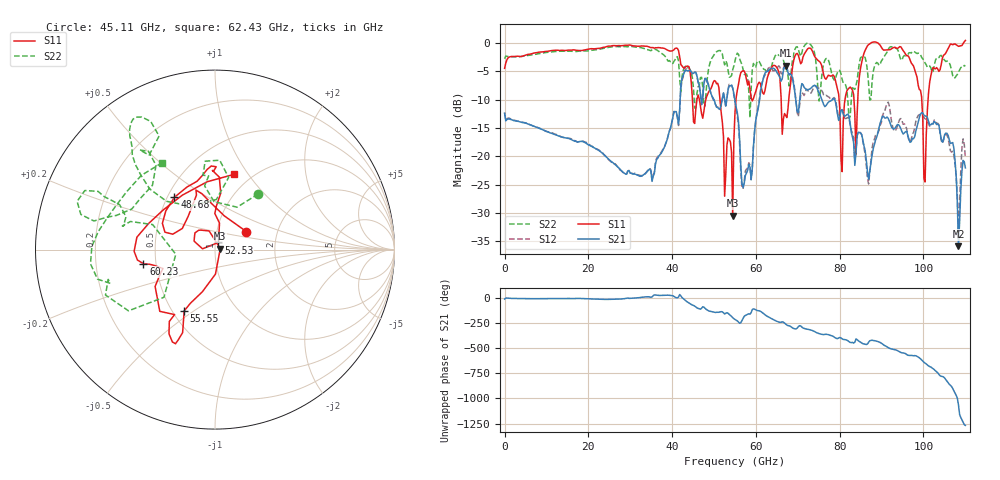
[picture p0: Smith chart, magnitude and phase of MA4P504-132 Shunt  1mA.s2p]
!Keysight Technologies,N5247B,US61255204,A.15.70.20
!Date: Friday, October 21, 2022 14:55:33
!Correction: S11(C  4-Port  )
!S31(C  4-Port  )
!S13(C  4-Port  )
!S33(C  4-Port  )
!S2P File: Measurements: S11, S31, S13, S33:
# Hz S  dB  R 50
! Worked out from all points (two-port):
!   401 points, 10 MHz to 110 GHz, reference 50 ohm
!   highest |S21| = -4.01 dB at 67.1 GHz (marker M1); lowest = -35.9 dB at 108.4 GHz (marker M2)
!   |S21| within 3 dB of the highest: 42.16 GHz to 46.25 GHz (4.099 GHz wide, 9.27 % of centre); 61.52 GHz to 68.91 GHz (7.396 GHz wide, 11.3 % of centre)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
!   lowest |S11| = -30.5 dB at 54.46 GHz (marker M3), VSWR 1.06, Z = 53 + j0.577 ohm
!   |S11| at or under -10 dB: 46.51 GHz to 48.04 GHz (1.53 GHz wide, 3.24 % of centre); 51.43 GHz to 55.24 GHz (3.815 GHz wide, 7.15 % of centre); 66.02 GHz to 67.84 GHz (1.818 GHz wide, 2.72 % of centre)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
!   |S22| runs from -13.3 to 0.0 dB; largest |S21 - S12| = 0.24
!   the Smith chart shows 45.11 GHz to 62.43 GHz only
!   S11 on the Smith chart (normalised r, x): 45.11 GHz: 1.39, +0.29; 48.68 GHz: 0.54, +0.37; 52.53 GHz: 1.04, +0.08; 55.55 GHz: 0.57, -0.46; 60.23 GHz: 0.43, -0.08; 62.43 GHz: 0.84, +0.86
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1e7  -4.46 -176.7  -12.37 -9.5  -12.35 -9.4  -2.78 -176.8
1.843332e10  -1.32 118.1  -17.37 -4.3  -17.39 -4.2  -1.41 124.6
3.685665e10  -0.80 115.3  -19.92 26.5  -19.76 26.5  -1.47 122.2
4.51059e10  -13.92 29.9  -5.36 -73.2  -5.44 -72.3  -8.12 52.2
4.868058e10  -8.66 127.8  -7.49 -126.1  -7.33 -124.8  -4.64 134.9
5.253022e10  -27.05 64.0  -9.85 -158.4  -9.96 -158.7  -3.85 124.8
5.445505e10  -30.47 10.5  -7.92 165.1  -8.01 164.2  -4.71 160.9
5.5005e10  -12.19 -106.7  -10.21 146.9  -10.45 145.0  -3.19 166.7
5.555495e10  -8.34 -116.7  -12.29 133.1  -12.88 132.3  -1.79 160.7
5.72048e10  -4.93 -114.8  -24.77 178.9  -24.40 -170.9  -5.54 159.8
6.022952e10  -7.83 -168.8  -12.56 -122.3  -12.35 -117.7  -3.42 -165.8
6.242932e10  -7.27 75.6  -5.05 -174.0  -5.25 -167.8  -4.94 121.2
6.71039e10  -12.78 -42.0  -4.01 101.5  -3.69 101.8  -4.38 45.6
7.342832e10  -1.33 138.5  -7.74 37.7  -8.45 35.9  -0.67 108.4
8.112762e10  -10.66 -29.9  -12.95 -53.1  -13.26 -54.0  -7.15 -124.7
8.525225e10  -3.37 38.3  -16.14 -87.7  -16.25 -86.5  -2.45 -23.7
9.185165e10  -1.17 90.5  -13.78 -139.2  -11.12 -133.5  -0.79 83.8
9.872602e10  -7.41 152.7  -13.97 132.9  -12.79 132.5  -1.78 177.4
1.003759e11  -24.53 -50.1  -12.88 72.4  -13.36 74.0  -3.51 -155.5
1.036756e11  -5.00 -33.6  -14.52 -40.2  -14.42 -37.4  -2.55 -90.1
1.083502e11  -0.58 22.5  -35.87 14.7  -33.66 21.4  -5.14 -4.9
1.1e11  0.46 54.4  -22.05 170.9  -20.31 172.3  -4.07 16.7
